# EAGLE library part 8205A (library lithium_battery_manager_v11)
DUAL N-CHANNEL MOSFET The 8205A uses advanced trench technology to provide excellent RDS(ON), low gate charge and operation with gate voltages as low as 2.5V. This device is suitable for use as a Battery protection or in other Switching application.
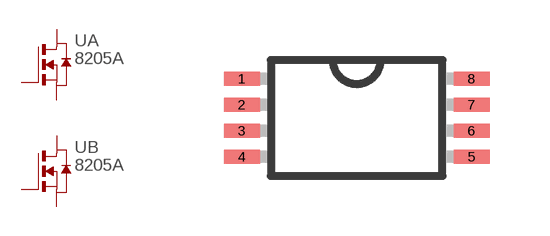
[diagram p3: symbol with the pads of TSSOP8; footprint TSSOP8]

Designator prefix -; gates A=N_MOSFET B=N_MOSFET

## 8205A  [TSSOP8]
1  A:D  pas
2  A:S  pas
3  A:S  pas
4  A:G  pas
5  B:G  pas
6  B:S  pas
7  B:S  pas
8  B:D  pas

## Footprint TSSOP8 (pad centres in mm)
8-Lead Thin Shrink Small Outline Package Source: http://www.analog.com/static/imported-files/data_sheets/AD8541_8542_8544.pdf
smd 0.9 x 0.35: 1 -2.875,0.975; 2 -2.875,0.325; 3 -2.875,-0.325; 4 -2.875,-0.975; 5 2.875,-0.975; 6 2.875,-0.325; 7 2.875,0.325; 8 2.875,0.975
